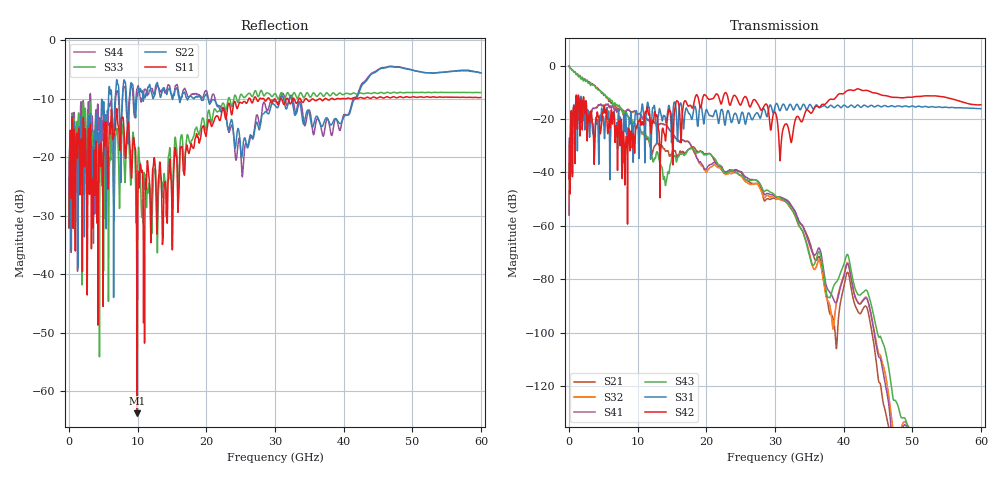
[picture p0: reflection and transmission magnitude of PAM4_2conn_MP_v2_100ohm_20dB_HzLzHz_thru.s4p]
! Info: Touchstone file created by Circ.  Input file=FAB50GbE_2conn_Midplane_Examax_Topo2_v2_100ohm_20dB_HzLzHz.circ
# Hz S RI R 50
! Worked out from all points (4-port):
!   6000 points, 10 MHz to 60 GHz, reference 50 ohm
!   strongest paths, dB at 10 MHz, 15.01 GHz, 30.01 GHz, 45.01 GHz, 60 GHz:
!     S42: -42.5, -25.2, -17.5, -10.5, -14.7
!     S31: -42.5, -23.5, -15.3, -14.9, -16.1
!     S43: -0.2, -33.5, -48.7, -100.9, -156.7
!     S41: -56.0, -25.1, -49.0, -108.2, -165.3
!     S32: -56.0, -25.2, -49.6, -107.0, -166.1
!     S21: -0.2, -32.7, -49.9, -116.6, -163.8
!   lowest |S11| = -63.8 dB at 9.92 GHz (marker M1), VSWR 1.00, Z = 50.1 + j0.0226 ohm
!   |S11| at or under -10 dB: start of sweep to 26.15 GHz; 34.61 GHz to 35.41 GHz (796.5 MHz wide, 2.28 % of centre); 35.54 GHz to 36.4 GHz (861.5 MHz wide, 2.4 % of centre)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
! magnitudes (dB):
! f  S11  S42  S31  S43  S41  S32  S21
! 10 MHz  -32.0  -42.5  -42.5  -0.2  -56.0  -56.0  -0.2
! 1.16 GHz  -17.0  -16.3  -17.7  -3.2  -21.2  -21.2  -3.1
! 9.92 GHz  -63.8  -22.3  -18.9  -22.7  -18.2  -17.9  -23.2
! 13.98 GHz  -24.2  -26.9  -19.1  -43.8  -22.0  -22.1  -31.7
! 31.7 GHz  -9.9  -21.9  -16.7  -51.1  -50.3  -51.4  -50.6
! 37.28 GHz  -9.9  -14.5  -15.1  -81.3  -79.9  -84.3  -83.4
! 60 GHz  -9.8  -14.7  -16.1  -156.7  -165.3  -166.1  -163.8
